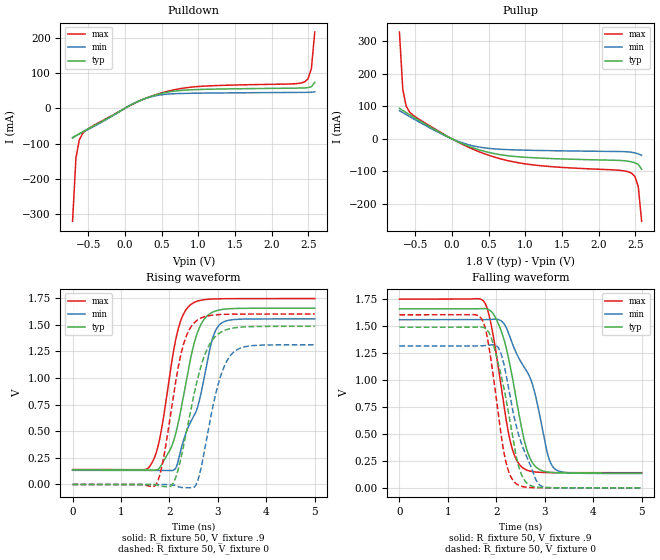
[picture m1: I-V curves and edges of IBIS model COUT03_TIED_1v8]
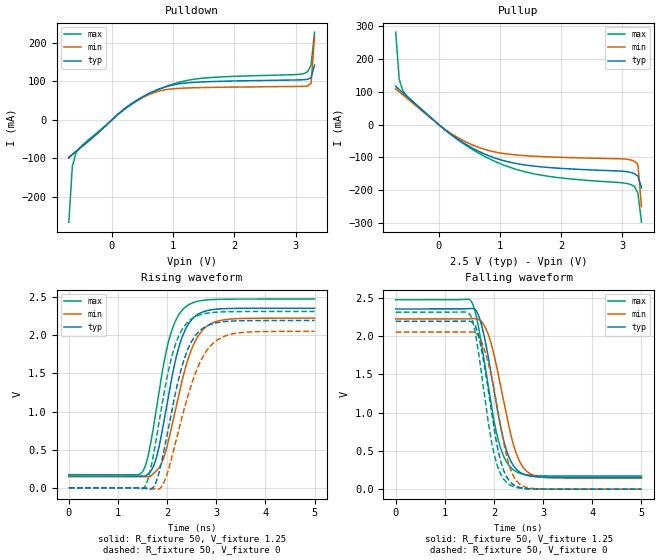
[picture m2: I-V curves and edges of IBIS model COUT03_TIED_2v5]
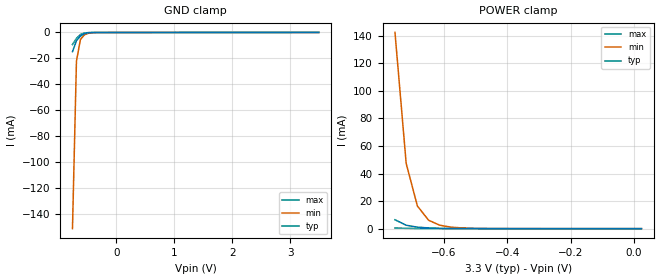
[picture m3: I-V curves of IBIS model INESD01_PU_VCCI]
|   This file is an IBIS representation of the   |
|   Integrated Device Technology , Inc.   |
|   ICS8305   |
|   LOW SKEW, 1-TO-4, MULTIPLEXED DIFF/LVCMOS-TO-LVCMOS/LVTTL FANOUT BUFFER   |
[IBIS Ver]   4.1
[File name]   8305.ibs
[File Rev]   1.1
[Date]   27 Oct 2010
|Rev 1.1 Oct 27, 2010
|Commented out the extreme currents in the clamps.
|Correlated the output buffer rt/ft to the lab data.
|Removed 2.5V input buffers.  This is a 3.3V VCC core only device,
|so inputs will only operate at 3.3V.
|(Outputs supports  VCCO of 1.8V, 2.5V, and 3.3V
|Rev 1.0  24 Nov 2009
|Updated model to IBIS 4.1
|Rev 0.0 May 23 2003
|Original Model
[Source]   Originated at Integrated Device Technology, Inc.
[Disclaimer]
IDT hereby grants the user of this IBIS model a non-exclusive,
nontransferable license to use this IBIS model under the following terms.
Before using this IBIS model, the user should read this license.
If the user does not accept these terms,  the IBIS model should be
returned to IDT within 30 days.
   The user is granted this license only to use the IBIS model and
is not granted rights to sell, load, rent, lease or license the IBIS
model in whole or in part, or in modified form to anyone other than
user. User may modify the IBIS model to suit its specific
applications but rights to derivative works and such modifications
shall belong to IDT.
   This IBIS model is provided on an "AS IS" basis and IDT makes
absolutely no warranty with respect to the information contained
herein. IDT DISCLAIMS AND CUSTOMER WAIVES ALL WARRANTIES, EXPRESS
OR IMPLIED, INCLUDING WARRANTIES OF MERCHANTABILITY OR FITNESS FOR
A PARTICULAR PURPOSE. The entire risk as to quality and performance
is with the Customer. ACCORDINGLY, IN NO EVENT SHALL THE COMPANY BE
LIABLE FOR ANY DAMAGES, WHETHER IN CONTRACT OR TORT,INCLUDING ANY
LOST PROFITS OR OTHER INCIDENTAL, CONSEQUENTIAL, EXEMPLARY, OR
PUNITIVE DAMAGES ARISING OUT OF THE USE OR APPLICATION OF THE IBIS
model provided in this package. Further, IDT reserves the right to
make changes without notice to any product herein to improve
reliability, function, or design. IDT does not convey any license
under patent rights or any other intellectual property rights,
including those of third parties.
   IDT is not obligated to provide maintenance or support
for the licensed IBIS model.
[Copyright]   Copyright 2003 by Integrated Device Technology , Inc.
[Component]   ICS8305
[Manufacturer] Integrated Device Technology, Inc.
[Package]
|   TSSOP16   typ   min   max
R_pkg   58.65m   52.5m   64.8m
L_pkg   1.902nH   1.443nH   2.361nH
C_pkg   0.315pF   0.254pF   0.375pF
[Pin] signal_name   model_name   R_pin   L_pin   C_pin
1   GND   GND   64.8m   2.361n   0.375p
2   OE   INESD01_PU_VCCI   60.7m   2.054n   0.335p
3   VDD   COUT03_TIED   56.6m   1.749n   0.294p
4   CLK_EN   INESD01_PU_VCCI   52.5m   1.443n   0.254p
5   CLK   INESD02_PD_VCCI   52.5m   1.443n   0.254p
6   nCLK   INESD02_PMID_VCC   56.6m   1.749n   0.294p
7   CLK_SEL   INESD01_PU_VCCI   60.7m   2.054n   0.335p
8   LVCMOS_CLK   INESD02_PD_VCCI   64.8m   2.361n   0.375p
9   GND   GND   64.8m   2.361n   0.375p
10   Q3   COUT03_TIED   60.7m   2.054n   0.335p
11   VDDO   POWER   56.6m   1.749n   0.294p
12   Q2   COUT03_TIED   52.5m   1.443n   0.254p
13   GND   GND   52.5m   1.443n   0.254p
14   Q1   COUT03_TIED   56.6m   1.749n   0.294p
15   VDDO   POWER   60.7m   2.054n   0.335p
16   QO   COUT03_TIED   64.8m   2.361n   0.375p
[Model Selector] COUT03_TIED
COUT03_TIED_1v8  Buffer selection for 1v8
COUT03_TIED_2v5  Buffer selection for 2v5
COUT03_TIED_3v3  Buffer selection for 3v3
| Models and submodels in the file (6): COUT03_TIED_1v8 (Output), COUT03_TIED_2v5 (Output), INESD01_PU_VCCI (Input), COUT03_TIED_3v3 (Output), INESD02_PD_VCCI (Input), INESD02_PMID_VCC (Input)
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[Model] COUT03_TIED_1v8
 Model_type   Output
Polarity   Non-Inverting
|   typ   min   max
C_comp   2pF   1.5pF   2.5pF
Vmeas = .9
Rref = 50
Cref = 0
Vref = .9
|   typ   min   max
[Voltage range]   1.8V   1.710V   1.890V
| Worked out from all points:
|   slope of the pulldown table from 0 to 0.27 V, typ, clamps not added: 9.89 ohm
|   slope of the pullup table from 0 to 0.27 V, typ, clamps not added: 10.2 ohm
|   rising waveform, R_fixture 50, V_fixture .9: 20-80 % time 419ps typ, 541ps min, 348ps max; typ from 0.136 V to 1.66 V
|   falling waveform, R_fixture 50, V_fixture .9: 20-80 % time 406ps typ, 617ps min, 343ps max; typ from 1.66 V to 0.136 V
|   rising waveform, R_fixture 50, V_fixture 0: 20-80 % time 444ps typ, 380ps min, 361ps max; typ from 0 V to 1.49 V
|   falling waveform, R_fixture 50, V_fixture 0: 20-80 % time 389ps typ, 453ps min, 304ps max; typ from 1.49 V to 0 V
[Pulldown]
|Voltage   I (typ)   I (min)   I (max)
|Note, modeling breaks down at 250mA and above.  This is well beyond the functional   |
|operating range of the device.  Should this scenario occur, catastrophic failure and   |
|possible damage to the device and/or board is of higher concern than the I-V curve   |
|behavior.  The IBIS checker will flag currents in excess of 10A with warnings.  Lines   |
|with currents in excess of 0.35 A have been commented out.  The points still remain|
|available to the user if the user desires to use them.   |
|-1.64000e+00   -9.54747e+00   -1.13153e+01   -8.54170e+00
|-1.48000e+00   -7.65574e+00   -8.67794e+00   -7.11904e+00
|-1.32000e+00   -5.76347e+00   -6.04044e+00   -5.69590e+00
|-1.16000e+00   -3.87057e+00   -3.40280e+00   -4.27240e+00
|-1.00000e+00   -1.97727e+00   -7.65056e-01   -2.84871e+00
|-9.90000e-01   -1.85893e+00   -6.00199e-01   -2.75973e+00
|-9.44138e-01   -1.31624e+00   -1.56449e-01   -2.35164e+00
|-8.98276e-01   -7.73592e-01   -1.08738e-01   -1.94356e+00
|-8.52414e-01   -2.71947e-01   -9.93900e-02   -1.53549e+00
|-8.06552e-01   -1.24502e-01   -9.33530e-02   -1.12747e+00
|-7.60690e-01   -9.45756e-02   -8.78175e-02   -7.19501e-01
-714.8mV  -84.49mA   -82.6mA    -320.1mA
-669mV    -77.89mA   -77.65mA   -141mA
-623.1mV  -72.09mA   -72.83mA   -89.45mA
-577.2mV  -66.62mA   -68.01mA   -71.44mA
-531.4mV  -61.39mA   -63.14mA   -62.41mA
110.7mV   12.63mA    13.07mA    12.2mA
477.6mV   40.96mA    37.72mA    42.28mA
982.1mV   53.05mA    42.74mA    61.38mA
2.45V     57.7mA     45.07mA    74.83mA
2.496V    58.55mA    45.16mA    83.48mA
2.541V    61.24mA    45.38mA    112.1mA
2.587V    73.4mA     46.71mA    216mA
| 2.63310e+00   1.40311e-01   6.02503e-02   6.01569e-01
| 2.67897e+00   5.31669e-01   2.19396e-01   1.22393e+00
| 2.72483e+00   1.36137e+00   1.21096e+00   1.84647e+00
| 2.77069e+00   2.19133e+00   2.37014e+00   2.46919e+00
| 2.81655e+00   3.02151e+00   3.52967e+00   3.09205e+00
| 2.86241e+00   3.85190e+00   4.68950e+00   3.71506e+00
| 2.90828e+00   4.68248e+00   5.84960e+00   4.33819e+00
| 2.95414e+00   5.51323e+00   7.00994e+00   4.96144e+00
| 3.00000e+00   6.34413e+00   8.17050e+00   5.58480e+00
| 3.01000e+00   6.52533e+00   8.42358e+00   5.72074e+00
| 3.12800e+00   8.66388e+00   1.14105e+01   7.32512e+00
| 3.24600e+00   1.08032e+01   1.43985e+01   8.93006e+00
| 3.36400e+00   1.29431e+01   1.73872e+01   1.05355e+01
| 3.48200e+00   1.50836e+01   2.03766e+01   1.21413e+01
| 3.60000e+00   1.72245e+01   2.33664e+01   1.37475e+01
[Pullup]
|Voltage   I (typ)   I (min)   I (max)
|Note, modeling breaks down at 250mA and above.  This is well beyond the functional   |
|operating range of the device.  Should this scenario occur, catastrophic failure and   |
|possible damage to the device and/or board is of higher concern than the I-V curve   |
|behavior.  The IBIS checker will flag currents in excess of 10A with warnings.  Lines   |
|with currents in excess of 0.35 A have been commented out.  The points still remain|
|available to the user if the user desires to use them.   |
|-1.64000e+00   1.44210e+01   1.71493e+01   1.28714e+01
|-1.48000e+00   1.15122e+01   1.30905e+01   1.06866e+01
|-1.32000e+00   8.60320e+00   9.03144e+00   8.50163e+00
|-1.16000e+00   5.69403e+00   4.97212e+00   6.31658e+00
|-1.00000e+00   2.78474e+00   9.12675e-01   4.13149e+00
|-9.90000e-01   2.60291e+00   6.58958e-01   3.99492e+00
|-9.44138e-01   1.76899e+00   1.61384e-01   3.36860e+00
|-8.98276e-01   9.35077e-01   1.14361e-01   2.74227e+00
|-8.52414e-01   2.78769e-01   1.04934e-01   2.11595e+00
|-8.06552e-01   1.33826e-01   9.86071e-02   1.48964e+00
|-7.60690e-01   1.04220e-01   9.25427e-02   8.63341e-01
-714.8mV  93.98mA    86.51mA    328.3mA
-669mV    87.01mA    80.49mA    152mA
-623.1mV  80.6mA     74.5mA     100.9mA
-531.4mV  68.07mA    62.6mA     73.05mA
110.7mV   -11.93mA   -9.872mA   -13.31mA
661mV     -48.79mA   -32.13mA   -61.34mA
1.166V    -58.87mA   -35.73mA   -81.67mA
2.266V    -66.3mA    -39.04mA   -96.44mA
2.45V     -70.88mA   -41.33mA   -105.7mA
2.496V    -73.74mA   -43.36mA   -115.8mA
2.541V    -78.71mA   -46.25mA   -146.4mA
2.587V    -93.41mA   -50.78mA   -253.5mA
| 2.63310e+00   -1.63849e-01   -6.79616e-02   -5.90488e-01
| 2.67897e+00   -5.27079e-01   -2.33405e-01   -9.96215e-01
| 2.72483e+00   -1.06768e+00   -9.51525e-01   -1.40213e+00
| 2.77069e+00   -1.60849e+00   -1.70633e+00   -1.80824e+00
| 2.81655e+00   -2.14948e+00   -2.46133e+00   -2.21449e+00
| 2.86241e+00   -2.69060e+00   -3.21648e+00   -2.62086e+00
| 2.90828e+00   -3.23185e+00   -3.97176e+00   -3.02734e+00
| 2.95414e+00   -3.77319e+00   -4.72713e+00   -3.43391e+00
| 3.00000e+00   -4.31462e+00   -5.48258e+00   -3.84056e+00
| 3.01000e+00   -4.43268e+00   -5.64731e+00   -3.92924e+00
| 3.12800e+00   -5.82608e+00   -7.59134e+00   -4.97585e+00
| 3.24600e+00   -7.21978e+00   -9.53562e+00   -6.02279e+00
| 3.36400e+00   -8.61367e+00   -1.14800e+01   -7.06994e+00
| 3.48200e+00   -1.00077e+01   -1.34245e+01   -8.11725e+00
| 3.60000e+00   -1.14018e+01   -1.53691e+01   -9.16466e+00
[Ramp]
|   typ   min   max
dV/dt_r   0.912/0.419n   0.856/0.542n   0.964/0.347n
dV/dt_f   0.914/0.407n   0.857/0.62n   0.967/0.344n
R_load =   50.0000
[Rising Waveform]
R_fixture = 50
V_fixture = .9   |Vcc_typ
V_fixture_min = .855 |Vcc_min
V_fixture_max = .945 |Vcc_max
C_fixture = 0.0p
| Time   typ   min   max
0s        136.4mV    132.9mV    140.2mV
1.592ns   136.4mV    132.9mV    169.1mV
1.797ns   155.2mV    133mV      424.4mV
2.067ns   383.7mV    131.9mV    1.208V
2.237ns   704mV      328.3mV    1.544V
2.457ns   1.228V     605.1mV    1.697V
2.693ns   1.537V     947.2mV    1.735V
2.883ns   1.618V     1.361V     1.743V
3.058ns   1.643V     1.511V     1.746V
5ns       1.657V     1.557V     1.747V
[Falling Waveform]
R_fixture = 50
V_fixture = .9   |Vcc_typ
V_fixture_min = .855 |Vcc_min
V_fixture_max = .945 |Vcc_max
C_fixture = 0.0p
| Time   typ   min   max
0s        1.657V     1.557V     1.747V
1.752ns   1.66V      1.557V     1.721V
1.912ns   1.626V     1.56V      1.468V
2.142ns   1.397V     1.529V     805.7mV
2.327ns   1.032V     1.339V     363.4mV
2.553ns   487.7mV    1.133V     183.1mV
2.783ns   209.8mV    899.2mV    148.1mV
3.058ns   146.3mV    314.1mV    141.4mV
3.203ns   140.1mV    177mV      140.7mV
5ns       136.4mV    132.9mV    140.2mV
[Rising Waveform]
R_fixture = 50
V_fixture = 0   |Vcc_typ
V_fixture_min = 0  |Vcc_min
V_fixture_max = 0 |Vcc_max
C_fixture = 0.0p
| Time   typ   min   max
0s        7.09nV     6.355nV    2.902uV
1.717ns   -3.767mV   35.98uV    -3.111mV
1.872ns   -18.62mV   408.4uV    232.2mV
2.117ns   50.37mV    -9.559mV   934.4mV
2.322ns   431.2mV    -30.01mV   1.363V
2.578ns   985.3mV    27.53mV    1.545V
2.773ns   1.266V     441.2mV    1.583V
2.993ns   1.41V      919.8mV    1.596V
3.273ns   1.467V     1.22V      1.601V
5ns       1.487V     1.313V     1.602V
[Falling Waveform]
R_fixture = 50
V_fixture = 0   |Vcc_typ
V_fixture_min = 0  |Vcc_min
V_fixture_max = 0 |Vcc_max
C_fixture = 0.0p
| Time   typ   min   max
0s        1.487V     1.313V     1.602V
1.697ns   1.489V     1.315V     1.564V
1.842ns   1.442V     1.32V      1.323V
2.077ns   1.083V     1.266V     560.3mV
2.227ns   758.1mV    985.7mV    190.3mV
2.417ns   279mV      562.2mV    35.91mV
2.603ns   57.82mV    314.1mV    6.647mV
2.818ns   7.502mV    74.44mV    1.02mV
2.933ns   2.588mV    15.32mV    402.8uV
5ns       12.39nV    347.4nV    2.896uV
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[Model] COUT03_TIED_2v5
Model_type   Output
Polarity   Non-Inverting
|   typ   min   max
C_comp   2pF   1.5pF   2.5pF
Vmeas = 1.25V
Rref = 50
Cref = 0
Vref = 1.25V
|   typ   min   max
[Voltage range]   2.5V   2.375V   2.625V
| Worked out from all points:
|   slope of the pulldown table from 0 to 0.375 V, typ, clamps not added: 7.84 ohm
|   slope of the pullup table from 0 to 0.375 V, typ, clamps not added: 7.16 ohm
|   rising waveform, R_fixture 50, V_fixture 1.25: 20-80 % time 418ps typ, 487ps min, 391ps max; typ from 0.154 V to 2.35 V
|   falling waveform, R_fixture 50, V_fixture 1.25: 20-80 % time 387ps typ, 425ps min, 376ps max; typ from 2.35 V to 0.154 V
|   rising waveform, R_fixture 50, V_fixture 0: 20-80 % time 463ps typ, 566ps min, 423ps max; typ from 0 V to 2.19 V
|   falling waveform, R_fixture 50, V_fixture 0: 20-80 % time 341ps typ, 378ps min, 332ps max; typ from 2.19 V to 0 V
[Pulldown]
|Voltage   I (typ)   I (min)   I (max)
|Note, modeling breaks down at 250mA and above.  This is well beyond the functional   |
|operating range of the device.  Should this scenario occur, catastrophic failure and   |
|possible damage to the device and/or board is of higher concern than the I-V curve   |
|behavior.  The IBIS checker will flag currents in excess of 10A with warnings.  Lines   |
|with currents in excess of 0.35 A have been commented out.  The points still remain|
|available to the user if the user desires to use them.   |
|-2.20000e+00   -1.62074e+01   -1.92448e+01   -1.35534e+01
|-1.90000e+00   -1.26590e+01   -1.47202e+01   -1.08842e+01
|-1.60000e+00   -9.10785e+00   -1.01942e+01   -8.21335e+00
|-1.30000e+00   -5.55419e+00   -5.66518e+00   -5.54094e+00
|-1.00000e+00   -1.99908e+00   -1.13389e+00   -2.86732e+00
|-9.90000e-01   -1.88056e+00   -9.82847e-01   -2.77818e+00
|-9.32644e-01   -1.20085e+00   -2.35159e-01   -2.26694e+00
|-8.75287e-01   -5.21184e-01   -1.26687e-01   -1.75571e+00
|-8.17931e-01   -1.60458e-01   -1.12537e-01   -1.24450e+00
|-7.60575e-01   -1.12013e-01   -1.04131e-01   -7.33346e-01
-703.2mV  -99.07mA   -96.45mA   -265.2mA
-645.9mV  -90.19mA   -89.16mA   -120.7mA
-588.5mV  -82.08mA   -82.01mA   -86.54mA
-473.8mV  -66.78mA   -67.48mA   -64.31mA
157.1mV   22.32mA    22.57mA    20.94mA
616mV     69.38mA    66.37mA    67.96mA
1.075V    93.01mA    81.56mA    96.53mA
1.534V    98.82mA    83.96mA    108.8mA
3.025V    103.6mA    86.77mA    117.6mA
3.197V    105.2mA    87.68mA    124.8mA
3.254V    109.7mA    95.12mA    142.6mA
3.312V    141.9mA    216.3mA    227.6mA
| 3.36908e+00   4.28521e-01   1.27896e+00   6.63452e-01
| 3.42644e+00   1.43728e+00   2.60453e+00   1.44187e+00
| 3.48379e+00   2.47535e+00   3.93059e+00   2.22057e+00
| 3.54115e+00   3.51378e+00   5.25706e+00   2.99953e+00
| 3.59851e+00   4.55252e+00   6.58390e+00   3.77872e+00
| 3.65586e+00   5.59154e+00   7.91106e+00   4.55812e+00
| 3.71322e+00   6.63082e+00   9.23852e+00   5.33770e+00
| 3.77057e+00   7.67033e+00   1.05662e+01   6.11747e+00
| 3.82793e+00   8.71005e+00   1.18942e+01   6.89740e+00
| 3.88529e+00   9.74997e+00   1.32224e+01   7.67748e+00
| 3.94264e+00   1.07901e+01   1.45508e+01   8.45771e+00
| 4.00000e+00   1.18303e+01   1.58793e+01   9.23807e+00
| 4.01000e+00   1.20117e+01   1.61110e+01   9.37414e+00
| 4.20800e+00   1.56041e+01   2.06988e+01   1.20691e+01
| 4.40600e+00   1.91982e+01   2.52885e+01   1.47654e+01
| 4.60400e+00   2.27940e+01   2.98802e+01   1.74631e+01
| 4.80200e+00   2.63917e+01   3.44742e+01   2.01624e+01
| 5.00000e+00   2.99918e+01   3.90710e+01   2.28635e+01
[Pullup]
|Voltage   I (typ)   I (min)   I (max)
|Note, modeling breaks down at 250mA and above.  This is well beyond the functional   |
|operating range of the device.  Should this scenario occur, catastrophic failure and   |
|possible damage to the device and/or board is of higher concern than the I-V curve   |
|behavior.  The IBIS checker will flag currents in excess of 10A with warnings.  Lines   |
|with currents in excess of 0.35 A have been commented out.  The points still remain|
|available to the user if the user desires to use them.   |
|-2.20000e+00   2.46568e+01   2.93416e+01   2.05715e+01
|-1.90000e+00   1.91989e+01   2.23786e+01   1.64695e+01
|-1.60000e+00   1.37396e+01   1.54140e+01   1.23669e+01
|-1.30000e+00   8.27894e+00   8.44769e+00   8.26356e+00
|-1.00000e+00   2.81709e+00   1.48000e+00   4.15967e+00
|-9.90000e-01   2.63501e+00   1.24772e+00   4.02286e+00
|-9.32644e-01   1.59065e+00   2.48527e-01   3.23819e+00
|-8.75287e-01   5.50231e-01   1.41619e-01   2.45351e+00
|-8.17931e-01   1.78662e-01   1.27107e-01   1.66881e+00
|-7.60575e-01   1.30328e-01   1.17885e-01   8.84116e-01
-703.2mV  116.7mA    108.9mA    281.4mA
-645.9mV  106.7mA    99.98mA    138.5mA
-588.5mV  97.11mA    91.01mA    103.8mA
-416.4mV  68.47mA    64.03mA    69.02mA
214.5mV   -31.81mA   -28.75mA   -32.68mA
730.7mV   -88.14mA   -74.48mA   -95.02mA
1.304V    -120mA     -93.16mA   -138.5mA
1.935V    -132.6mA   -99.35mA   -161.1mA
3.025V    -142.3mA   -104.7mA   -177.9mA
3.197V    -149.5mA   -111.7mA   -188.9mA
3.254V    -156.9mA   -122.9mA   -208.7mA
3.312V    -192.7mA   -250mA     -297.2mA
| 3.36908e+00   -4.86496e-01   -1.03142e+00   -6.80808e-01
| 3.42644e+00   -1.16265e+00   -1.89462e+00   -1.18836e+00
| 3.48379e+00   -1.83911e+00   -2.75813e+00   -1.69622e+00
| 3.54115e+00   -2.51584e+00   -3.62188e+00   -2.20432e+00
| 3.59851e+00   -3.19276e+00   -4.48581e+00   -2.71263e+00
| 3.65586e+00   -3.86984e+00   -5.34989e+00   -3.22109e+00
| 3.71322e+00   -4.54706e+00   -6.21408e+00   -3.72969e+00
| 3.77057e+00   -5.22438e+00   -7.07837e+00   -4.23841e+00
| 3.82793e+00   -5.90178e+00   -7.94273e+00   -4.74723e+00
| 3.88529e+00   -6.57926e+00   -8.80714e+00   -5.25612e+00
| 3.94264e+00   -7.25679e+00   -9.67161e+00   -5.76509e+00
| 4.00000e+00   -7.93437e+00   -1.05361e+01   -6.27411e+00
| 4.01000e+00   -8.05251e+00   -1.06868e+01   -6.36286e+00
| 4.20800e+00   -1.03918e+01   -1.36714e+01   -8.12040e+00
| 4.40600e+00   -1.27313e+01   -1.66560e+01   -9.87821e+00
| 4.60400e+00   -1.50709e+01   -1.96407e+01   -1.16361e+01
| 4.80200e+00   -1.74104e+01   -2.26254e+01   -1.33941e+01
| 5.00000e+00   -1.97499e+01   -2.56100e+01   -1.51520e+01
[Ramp]
|   typ   min   max
dV/dt_r   1.321/0.418n   1.249/0.487n   1.382/0.391n
dV/dt_f   1.324/0.388n   1.251/0.426n   1.387/0.377n
R_load =   50.0000
[Rising Waveform]
R_fixture = 50
V_fixture = 1.25   |Vcc_typ
V_fixture_min = 1.1875 |Vcc_min
V_fixture_max = 1.3125 |Vcc_max
C_fixture = 0.0p
| Time   typ   min   max
0s        154.1mV    144.1mV    172.2mV
1.502ns   152.6mV    144.3mV    211.3mV
1.607ns   177.2mV    143mV      401.1mV
1.727ns   287.6mV    188.7mV    811.3mV
1.907ns   771.2mV    350.6mV    1.54V
2.122ns   1.531V     887.1mV    2.114V
2.402ns   2.114V     1.639V     2.386V
2.653ns   2.285V     2.012V     2.45V
2.983ns   2.342V     2.177V     2.471V
5ns       2.355V     2.225V     2.475V
[Falling Waveform]
R_fixture = 50
V_fixture = 1.25   |Vcc_typ
V_fixture_min = 1.1875 |Vcc_min
V_fixture_max = 1.3125 |Vcc_max
C_fixture = 0.0p
| Time   typ   min   max
0s        2.355V     2.225V     2.475V
1.537ns   2.362V     2.228V     2.454V
1.702ns   2.24V      2.214V     2.061V
1.902ns   1.66V      1.988V     1.263V
2.132ns   822.1mV    1.357V     542.4mV
2.262ns   492.5mV    944.8mV    349.4mV
2.402ns   300.7mV    567.3mV    248.8mV
2.593ns   197.6mV    286.3mV    196.1mV
2.863ns   161.5mV    169.2mV    176.7mV
5ns       154.1mV    144.1mV    172.2mV
[Rising Waveform]
R_fixture = 50
V_fixture   =0
V_fixture_min =0
V_fixture_max =0
C_fixture = 0.0p
| Time   typ   min   max
0s        7.212nV    6.502nV    4.144uV
1.542ns   -7.567mV   -17.71uV   10.27mV
1.637ns   -17.66mV   -6.8mV     174.2mV
1.752ns   40.24mV    -16.44mV   537.4mV
1.937ns   489.6mV    72.33mV    1.24V
2.182ns   1.279V     621.7mV    1.904V
2.492ns   1.912V     1.351V     2.212V
2.783ns   2.115V     1.778V     2.287V
3.138ns   2.178V     1.98V      2.308V
5ns       2.194V     2.052V     2.313V
[Falling Waveform]
R_fixture = 50
V_fixture   =0
V_fixture_min =0
V_fixture_max =0
C_fixture = 0.0p
| Time   typ   min   max
0s        2.194V     2.052V     2.313V
1.512ns   2.193V     2.055V     2.28V
1.597ns   2.158V     2.049V     2.114V
1.707ns   1.943V     1.983V     1.691V
1.997ns   816mV      1.315V     474mV
2.137ns   364mV      813.7mV    196.2mV
2.297ns   120.4mV    334.9mV    66.12mV
2.462ns   35.29mV    105.1mV    20.85mV
2.708ns   5.471mV    15.92mV    3.708mV
5ns       569.6pV    556pV      4.137uV
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[Model] INESD01_PU_VCCI
Model_type   Input
Polarity   Non-Inverting
Vinl = 0.8V
Vinh = 2.0V
|   typ   min   max
C_comp   2pF   1.5pF   2.5pF
|   typ   min   max
[Voltage range]   3.3V   3.135V   3.465V
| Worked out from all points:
|   GND clamp passes 1 mA (typ) near -0.55 V on its own axis
|   POWER clamp passes 1 mA (typ) near -0.68 V on its own axis
[GND_clamp]
|Voltage   I (typ)   I (min)   I (max)
|Note, modeling breaks down at 250mA and above.  This is well beyond the functional   |
|operating range of the device.  Should this scenario occur, catastrophic failure and   |
|possible damage to the device and/or board is of higher concern than the I-V curve   |
|behavior.  The IBIS checker will flag currents in excess of 10A with warnings.  Lines   |
|with currents in excess of 0.35 A have been commented out.  The points still remain|
|available to the user if the user desires to use them.   |
|-3.30000e+00   -2.90479e+01   -2.50897e+01   -3.57066e+01
|-3.23131e+00   -2.82366e+01   -2.44134e+01   -3.46710e+01
|-3.16263e+00   -2.74254e+01   -2.37370e+01   -3.36354e+01
|-3.09394e+00   -2.66141e+01   -2.30607e+01   -3.25999e+01
|-3.02525e+00   -2.58028e+01   -2.23843e+01   -3.15643e+01
|-2.95657e+00   -2.49915e+01   -2.17080e+01   -3.05287e+01
|-2.88788e+00   -2.41802e+01   -2.10316e+01   -2.94932e+01
|-2.81919e+00   -2.33690e+01   -2.03553e+01   -2.84576e+01
|-2.75051e+00   -2.25577e+01   -1.96790e+01   -2.74220e+01
|-2.68182e+00   -2.17464e+01   -1.90027e+01   -2.63864e+01
|-2.61313e+00   -2.09351e+01   -1.83263e+01   -2.53508e+01
|-2.54444e+00   -2.01238e+01   -1.76500e+01   -2.43152e+01
|-2.47576e+00   -1.93126e+01   -1.69737e+01   -2.32795e+01
|-2.40707e+00   -1.85013e+01   -1.62974e+01   -2.22439e+01
|-2.33838e+00   -1.76900e+01   -1.56211e+01   -2.12082e+01
|-2.26970e+00   -1.68787e+01   -1.49448e+01   -2.01726e+01
|-2.20101e+00   -1.60674e+01   -1.42686e+01   -1.91369e+01
|-2.13232e+00   -1.52561e+01   -1.35923e+01   -1.81012e+01
|-2.06364e+00   -1.44448e+01   -1.29160e+01   -1.70654e+01
|-1.99495e+00   -1.36335e+01   -1.22398e+01   -1.60297e+01
|-1.92626e+00   -1.28221e+01   -1.15636e+01   -1.49939e+01
|-1.85758e+00   -1.20109e+01   -1.08874e+01   -1.39582e+01
|-1.78889e+00   -1.11996e+01   -1.02112e+01   -1.29224e+01
|-1.72020e+00   -1.03883e+01   -9.53505e+00   -1.18866e+01
|-1.65152e+00   -9.57705e+00   -8.85895e+00   -1.08508e+01
|-1.58283e+00   -8.76583e+00   -8.18290e+00   -9.81502e+00
|-1.51414e+00   -7.95465e+00   -7.50691e+00   -8.77924e+00
|-1.44545e+00   -7.14353e+00   -6.83099e+00   -7.74348e+00
|-1.37677e+00   -6.33247e+00   -6.15516e+00   -6.70775e+00
|-1.30808e+00   -5.52151e+00   -5.47943e+00   -5.67207e+00
|-1.23939e+00   -4.71065e+00   -4.80384e+00   -4.63647e+00
|-1.17071e+00   -3.89994e+00   -4.12840e+00   -3.60097e+00
|-1.10202e+00   -3.08942e+00   -3.45315e+00   -2.56562e+00
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-758.6mV  -14.85mA   -150.9mA   -9.33mA
-689.9mV  -6.314mA   -22.17mA   -4.562mA
-621.2mV  -2.834mA   -5.461mA   -1.625mA
-552.5mV  -1.021mA   -1.876mA   -431.7uA
-483.8mV  -316uA     -644uA     -125.2uA
-346.5mV  -78.62uA   -116.7uA   -58.21uA
3.5V      3.9uA      19.39uA    528.4nA
[Power_clamp]
|Voltage   I (typ)   I (min)   I (max)
|Note, modeling breaks down at 250mA and above.  This is well beyond the functional   |
|operating range of the device.  Should this scenario occur, catastrophic failure and   |
|possible damage to the device and/or board is of higher concern than the I-V curve   |
|behavior.  The IBIS checker will flag currents in excess of 10A with warnings.  Lines   |
|with currents in excess of 0.35 A have been commented out.  The points still remain|
|available to the user if the user desires to use them.   |
|-3.30000e+00   5.07435e+01   4.37800e+01   6.24704e+01
|-3.26465e+00   5.00098e+01   4.31687e+01   6.15331e+01
|-3.22929e+00   4.92761e+01   4.25574e+01   6.05959e+01
|-3.19394e+00   4.85424e+01   4.19461e+01   5.96587e+01
|-3.15859e+00   4.78087e+01   4.13348e+01   5.87215e+01
|-3.12323e+00   4.70751e+01   4.07235e+01   5.77842e+01
|-3.08788e+00   4.63414e+01   4.01123e+01   5.68470e+01
|-3.05253e+00   4.56077e+01   3.95010e+01   5.59098e+01
|-3.01717e+00   4.48741e+01   3.88897e+01   5.49726e+01
|-2.98182e+00   4.41404e+01   3.82785e+01   5.40353e+01
|-2.94646e+00   4.34068e+01   3.76673e+01   5.30981e+01
|-2.91111e+00   4.26732e+01   3.70560e+01   5.21609e+01
|-2.87576e+00   4.19395e+01   3.64448e+01   5.12236e+01
|-2.84040e+00   4.12059e+01   3.58336e+01   5.02864e+01
|-2.80505e+00   4.04723e+01   3.52225e+01   4.93492e+01
|-2.76970e+00   3.97387e+01   3.46113e+01   4.84119e+01
|-2.73434e+00   3.90050e+01   3.40001e+01   4.74747e+01
|-2.69899e+00   3.82714e+01   3.33890e+01   4.65375e+01
|-2.66364e+00   3.75378e+01   3.27778e+01   4.56003e+01
|-2.62828e+00   3.68043e+01   3.21667e+01   4.46630e+01
|-2.59293e+00   3.60707e+01   3.15556e+01   4.37258e+01
|-2.55758e+00   3.53371e+01   3.09445e+01   4.27886e+01
|-2.52222e+00   3.46036e+01   3.03334e+01   4.18514e+01
|-2.48687e+00   3.38700e+01   2.97223e+01   4.09142e+01
|-2.45152e+00   3.31365e+01   2.91112e+01   3.99770e+01
|-2.41616e+00   3.24029e+01   2.85002e+01   3.90398e+01
|-2.38081e+00   3.16694e+01   2.78891e+01   3.81026e+01
|-2.34545e+00   3.09359e+01   2.72781e+01   3.71654e+01
|-2.31010e+00   3.02024e+01   2.66671e+01   3.62282e+01
|-2.27475e+00   2.94689e+01   2.60561e+01   3.52910e+01
|-2.23939e+00   2.87355e+01   2.54452e+01   3.43539e+01
|-2.20404e+00   2.80020e+01   2.48342e+01   3.34167e+01
|-2.16869e+00   2.72686e+01   2.42233e+01   3.24796e+01
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-754.5mV  6.457mA    142.4mA    482.6uA
-719.2mV  2.486mA    47.33mA    227.8uA
-683.8mV  1.109mA    16.45mA    105.9uA
-648.5mV  532.4uA    6.125mA    50.08uA
-613.1mV  259.9uA    2.485mA    25.29uA
-542.4mV  63.18uA    506.4uA    10.19uA
23.23mV   -452.4nA   -560.5nA   -350.7nA
